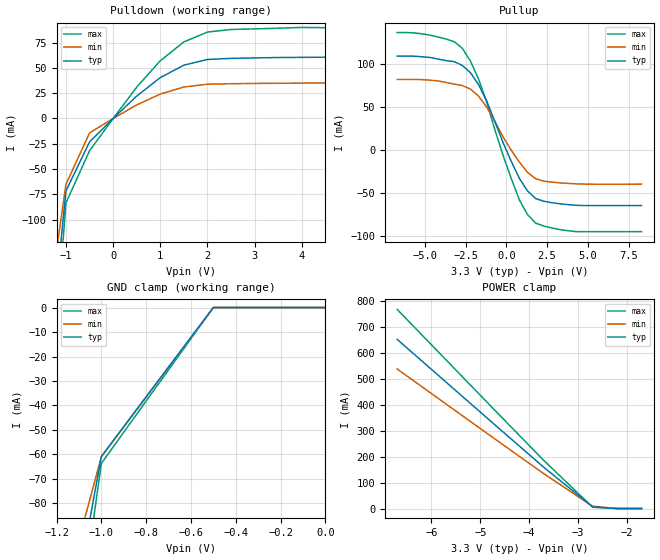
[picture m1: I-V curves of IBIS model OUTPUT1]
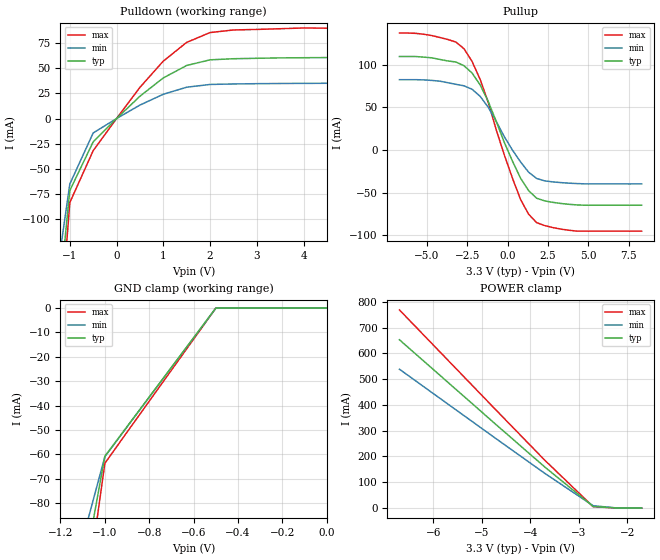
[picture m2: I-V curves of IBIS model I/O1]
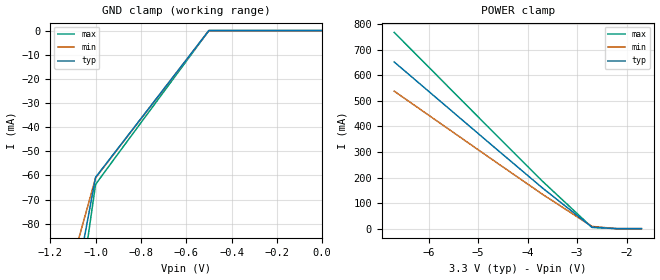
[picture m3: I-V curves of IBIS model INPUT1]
[IBIS Ver]   1.1
[File name]   960hxpq2.ibs
[File rev]   1.0
[Date]   5/10/96
[Source]   The file was oringinated at Intel Corporation.
[Notes]   The following information corresponds to the 80960HA
   in the 168 lead PGA package. This information has
   not been correlated to actual silicon.
[Disclaimer]   This information is for modeling purposes only and is
   not guaranteed.
[Component]   80960HX
[Manufacturer]  Intel
[Package]PQ@
|	typ   min   max
R_pkg	130m	117m	145m
L_pkg	12.4nH	10.9nH	13.9nH
C_pkg	1.1pF	.9pF	1.3pF
[Pin]   signal_name   model_name
A1	VSS		GND
A2	FAIL#		OUTPUT1
A3	DP0		I/O1
A4	DP2		I/O1
A5	VOLDET		OUTPUT1
A6	TRST		INPUT1
A7	TDI		INPUT1
A8	TDO		OUTPUT1
A9	NC		NC
A10	NC		NC
A11	CT0		OUTPUT1
A12	CT1		OUTPUT1
A13	CT2		OUTPUT1
A14	CT3		OUTPUT1
A15	XINT1#		INPUT1
A16	RESET#		RSTBUF
A17	XINT2#		INPUT1
B1	BOFF#		INPUT1
B2	STEST		INPUT1
B3	DP1		I/O1
B4	DP3		I/O1
B5	TCK		INPUT1
B6	TMS		INPUT1
B7	VCC		POWER
B8	PCHK#		OUTPUT1
B9	VCC		POWER
B10	VCCPLL		INPUT1
B11	VCC		POWER
B12	VCC		POWER
B13	NC		NC
B14	NC		NC
B15	XINT0#		INPUT1
B16	XINT3#		INPUT1
B17	XINT5#		INPUT1
C1	D3		I/O1
C2	D1		I/O1
C3	ONCE#		INPUT1
C4	VSS		GND
C5	VCC5		INPUT1
C6	VCC		POWER
C7	VSS		GND
C8	VSS		GND
C9	VSS		GND
C10	VSS		GND
C11	VSS		GND
C12	VSS		GND
C13	CLKIN		CLKBUF
C14	VSS		GND
C15	XINT4#		INPUT1
C16	XINT6#		INPUT1
C17	XINT7#		INPUT1
D1	D5		I/O1
D2	D2		I/O1
D3	NC		NC
D15	NMI#		INPUT1
D16	A2		OUTPUT1
D17	A3		OUTPUT1
E1	D7		I/O1
E2	D4		I/O1
E3	D0		I/O1
E15	VCC		POWER
E16	A4		OUTPUT1
E17	A5		OUTPUT1
F1	D8		I/O1
F2	D6		I/O1
F3	VCC		POWER
F15	VSS		GND
F16	VCC		POWER
F17	A6		OUTPUT1
G1	D9		I/O1
G2	VCC		POWER
G3	VSS		GND
G15	VSS		GND
G16	A7		OUTPUT1
G17	A8		OUTPUT1
H1	D11		I/O1
H2	D10		I/O1
H3	VSS		GND
H15	VSS		GND
H16	VCC		POWER
H17	A9		OUTPUT1
J1	D12		I/O1
J2	VCC		POWER
J3	VSS		GND
J15	VSS		GND
J16	VCC		POWER
J17	A10		OUTPUT1
K1	D13		I/O1
K2	VCC		POWER
K3	VSS		GND
K15	VSS		GND
K16	VCC		POWER
K17	A11		OUTPUT1
L1	D15		I/O1
L2	D14		I/O1
L3	VSS		GND
L15	VSS		GND
L16	A13		OUTPUT1
L17	A12		OUTPUT1
M1	D16		I/O1
M2	VCC		POWER
M3	VSS		GND
M15	VSS		GND
M16	VCC		POWER
M17	A14		OUTPUT1
N1	D17		I/O1
N2	D18		I/O1
N3	VCC		POWER
N15	VCC		POWER
N16	A16		OUTPUT1
N17	A15		OUTPUT1
P1	A19		OUTPUT1
P2	D20		I/O1
P3	D22		I/O1
P15	A20		OUTPUT1
P16	A19		OUTPUT1
P17	A17		OUTPUT1
Q1	D21		I/O1
Q2	D23		I/O1
Q3	D26		I/O1
Q4	D28		I/O1
Q5	D30		I/O1
Q6	VCC		POWER
Q7	VSS		GND
Q8	VSS		GND
Q9	VSS		GND
Q10	VSS		GND
Q11	VSS		GND
Q12	SUP#		OUTPUT1
Q13	A30		OUTPUT1
Q14	A28		OUTPUT1
Q15	A24		OUTPUT1
Q16	A21		OUTPUT1
Q17	A18		OUTPUT1
R1	D24		I/O1
R2	D27		I/O1
R3	D31		I/O1
R4	BTERM#		INPUT1
R5	HOLD		INPUT1
R6	ADS#		OUTPUT1
R7	VCC		POWER
R8	VCC		POWER
R9	BE0#		OUTPUT1
R10	VCC		POWER
R11	VCC		POWER
R12	BSTALL		OUTPUT1
R13	BREQ		OUTPUT1
R14	A29		OUTPUT1
R15	A26		OUTPUT1
R16	A23		OUTPUT1
R17	A22		OUTPUT1
S1	D25		I/O1
S2	D29		I/O1
S3	READY#		INPUT1
S4	HOLDA		OUTPUT1
S5	BE3#		OUTPUT1
S6	BE2#		OUTPUT1
S7	BE1#		OUTPUT1
S8	BLAST#		OUTPUT1
S9	DEN#		OUTPUT1
S10	W/R#		OUTPUT1
S11	DT#/R#		OUTPUT1
S12	WAIT#		OUTPUT1
S13	D#/C#		OUTPUT1
S14	LOCK#		OUTPUT1
S15	A31		OUTPUT1
S16	A27		OUTPUT1
S17	A25		OUTPUT1
| Models and submodels in the file (5): OUTPUT1 (Output), I/O1 (I/O), INPUT1 (Input), CLKBUF (Input), RSTBUF (Input)
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|This following model descriptions describe each of the
|different type of buffers.
|This is the model for buffer OUTPUT1.
[Model] OUTPUT1
Model_type Output
Polarity Non-Inverting
Enable Active-High
|signals  FAIL#,VOLDET,CT(3:0),PCHK#,A(31:2),SUP#,ADS#,BE(3:0)#,BSTALL,
|   BREQ,HOLDA,BLAST#,DEN#,W/R#,DT#/R#,WAIT#,D#/C#,LOCK#,TDO
|variable   typ   min   max
C_comp   3.2pf	2.9pf	3.5pf
|variable   typ   min   max
[Voltage range]   3.3V   3.0V   3.6V
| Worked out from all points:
|   slope of the pulldown table from 0 to 0.495 V, typ, clamps not added: 22.6 ohm
|   slope of the pullup table from 0 to 0.495 V, typ, clamps not added: 23.8 ohm
|   GND clamp passes 1 mA (typ) near -0.51 V on its own axis
|   POWER clamp passes 1 mA (typ) near -2.28 V on its own axis
[Pulldown]
|Voltage   I(typ)   I(min)   I(max)
-5V       -2.148A    -1.467A    -2.772A
-1.5V     -307.3mA   -227.6mA   -382.9mA
-1V       -71.49mA   -65.01mA   -83.39mA
-500mV    -23.17mA   -14.29mA   -31.92mA
500mV     22.15mA    13.38mA    30.94mA
1V        40.34mA    24.11mA    57.02mA
1.5V      52.68mA    31.12mA    75.61mA
2V        58.31mA    33.86mA    85.36mA
2.5V      59.38mA    34.34mA    87.93mA
4V        60.39mA    34.93mA    89.94mA
10V       60.77mA    35.16mA    90.06mA
|Note that the pullup voltage in the data table is derived from the
|equation:
|Vtable = Vcc - Voutput
|For the 8.3V in the table it is actually 8.3 volts below Vcc and
|-3.3V with respect to ground.
[Pullup]
|Voltage   I(typ)   I(min)   I(max)
-6.7V     109.6mA    82.49mA    137.1mA
-4.2V     106.2mA    80.75mA    131.9mA
-3.2V     103.2mA    77.06mA    126.5mA
-2.7V     98.79mA    75.33mA    118.7mA
-1.7V     76.29mA    62.98mA    82.73mA
-1.2V     57mA       50.13mA    55.93mA
-200mV    8.81mA     15.56mA    -5.959mA
800mV     -32.82mA   -13.78mA   -57.82mA
1.3V      -47.47mA   -25.86mA   -75.07mA
1.8V      -56.38mA   -33.22mA   -84.96mA
4.3V      -64.2mA    -39.19mA   -94.9mA
8.3V      -64.54mA   -39.59mA   -94.91mA
[GND_Clamp]
|Voltage   I(typ)   I(min)   I(max)
-5V       -2.148A    -1.466A    -2.772A
-2V       -564.4mA   -400.4mA   -716.6mA
-1V       -60.81mA   -61.01mA   -63.72mA
-900mV    -48.65mA   -48.79mA   -50.93mA
-800mV    -36.49mA   -36.6mA    -38.2mA
-700mV    -24.32mA   -24.4mA    -25.46mA
-600mV    -12.16mA   -12.2mA    -12.73mA
-500mV    0A         0A         0A
-400mV    0A         0A         0A
0V        0A         0A         0A
|Note that the voltages in the Power_clamp data table are Vcc relative
|which means they are referenced to Vcc.  The voltages in the table are
|derived from the following equation:
|Vtable = Vcc - Voutput
|0V in the table is actually 3.3V with respect to ground and 0V above Vcc.
[POWER_Clamp]
|Voltage   I(typ)   I(min)   I(max)
-6.7V     652.6mA    538.3mA    768.3mA
-4.7V     322.7mA    268.2mA    378.8mA
-3.7V     159.1mA    134.5mA    185.5mA
-2.7V     6mA        8.856mA    4.991mA
-2.6V     4.8mA      7.109mA    3.988mA
-2.5V     3.6mA      5.338mA    2.997mA
-2.4V     2.4mA      3.559mA    1.994mA
-2.3V     1.2mA      1.779mA    1.003mA
-2.2V     0A         0A         0A
-1.7V     0A         0A         0A
[Ramp]
|   typ   min   max
dV/dt_r   1.3/0.3n	1.1/0.5n	1.5/0.3n
dV/dt_f		1.3/0.3n	1.0/0.5n	1.5/0.3n
|end of OUTPUT1 model
|This is the model for the buffer I/O1.
[Model] I/O1
Model_type I/O
Polarity Non-Inverting
Enable Active-High
|Signals  D(31:0),DP(3:0)
Vinl = 0.8V
Vinh = 2.0V
|variable   typ   min   max
C_comp   3.2pf	2.9pf	3.5pf
|variable   typ   min   max
[Voltage range]   3.3V   3.0V   3.6V
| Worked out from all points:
|   slope of the pulldown table from 0 to 0.495 V, typ, clamps not added: 22.6 ohm
|   slope of the pullup table from 0 to 0.495 V, typ, clamps not added: 23.8 ohm
|   GND clamp passes 1 mA (typ) near -0.51 V on its own axis
|   POWER clamp passes 1 mA (typ) near -2.28 V on its own axis
[Pulldown]
|Voltage   I(typ)   I(min)   I(max)
-5V       -2.148A    -1.467A    -2.772A
-1.5V     -307.3mA   -227.6mA   -382.9mA
-1V       -71.49mA   -65.01mA   -83.39mA
-500mV    -23.17mA   -14.29mA   -31.92mA
500mV     22.15mA    13.38mA    30.94mA
1V        40.34mA    24.11mA    57.02mA
1.5V      52.68mA    31.12mA    75.61mA
2V        58.31mA    33.86mA    85.36mA
2.5V      59.38mA    34.34mA    87.93mA
4V        60.39mA    34.93mA    89.94mA
10V       60.77mA    35.16mA    90.06mA
|Note that the pullup voltage in the data table is derived from the
|equation:
|Vtable = Vcc - Voutput
|For the 8.3V in the table it is actually 8.3 volts below Vcc and
|-3.3V with respect to ground.
[Pullup]
|Voltage   I(typ)   I(min)   I(max)
-6.7V     109.6mA    82.49mA    137.1mA
-4.2V     106.2mA    80.75mA    131.9mA
-3.2V     103.2mA    77.06mA    126.5mA
-2.7V     98.79mA    75.33mA    118.7mA
-1.7V     76.29mA    62.98mA    82.73mA
-1.2V     57mA       50.13mA    55.93mA
-200mV    8.81mA     15.56mA    -5.959mA
800mV     -32.82mA   -13.78mA   -57.82mA
1.3V      -47.47mA   -25.86mA   -75.07mA
1.8V      -56.38mA   -33.22mA   -84.96mA
4.3V      -64.2mA    -39.19mA   -94.9mA
8.3V      -64.54mA   -39.59mA   -94.91mA
[GND_Clamp]
|Voltage   I(typ)   I(min)   I(max)
-5V       -2.148A    -1.466A    -2.772A
-2V       -564.4mA   -400.4mA   -716.6mA
-1V       -60.81mA   -61.01mA   -63.72mA
-900mV    -48.65mA   -48.79mA   -50.93mA
-800mV    -36.49mA   -36.6mA    -38.2mA
-700mV    -24.32mA   -24.4mA    -25.46mA
-600mV    -12.16mA   -12.2mA    -12.73mA
-500mV    0A         0A         0A
-400mV    0A         0A         0A
0V        0A         0A         0A
|Note that the voltages in the Power_clamp data table are Vcc relative
|which means they are referenced to Vcc.  The voltages in the table are
|derived from the following equation:
|Vtable = Vcc - Voutput
|0V in the table is actually 3.3V with respect to ground and 0V above Vcc.
[POWER_Clamp]
|Voltage   I(typ)   I(min)   I(max)
-6.7V     652.6mA    538.3mA    768.3mA
-4.7V     322.7mA    268.2mA    378.8mA
-3.7V     159.1mA    134.5mA    185.5mA
-2.7V     6mA        8.856mA    4.991mA
-2.6V     4.8mA      7.109mA    3.988mA
-2.5V     3.6mA      5.338mA    2.997mA
-2.4V     2.4mA      3.559mA    1.994mA
-2.3V     1.2mA      1.779mA    1.003mA
-2.2V     0A         0A         0A
-1.7V     0A         0A         0A
[Ramp]
|   typ   min   max
dV/dt_r   1.3/0.3n	1.1/0.5n	1.5/0.3n
dV/dt_f		1.3/0.3n	1.0/0.5n	1.5/0.3n
|end of I/O1 model
|This is the model for the buffer INPUT1.
[Model] INPUT1
Model_type Input
Polarity Non-Inverting
Enable Active-High
|Signals  TRST,TDI,XINT(7:0)#,BOFF#,STEST,TCK,TMS,VCCPLL,ONCE#,
|	  VCC5,NMI#,BTERM#,HOLD,READY#
Vinl = 0.8V
Vinh = 2.0V
|variable   typ   min   max
C_comp   3.2pf	2.9pf	3.5pf
|variable   typ   min   max
[Voltage range]   3.3V   3.0V   3.6V
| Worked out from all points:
|   GND clamp passes 1 mA (typ) near -0.51 V on its own axis
|   POWER clamp passes 1 mA (typ) near -2.28 V on its own axis
[GND_Clamp]
|Voltage   I(typ)   I(min)   I(max)
-5V       -2.148A    -1.466A    -2.772A
-2V       -564.4mA   -400.4mA   -716.6mA
-1V       -60.81mA   -61.01mA   -63.72mA
-900mV    -48.65mA   -48.79mA   -50.93mA
-800mV    -36.49mA   -36.6mA    -38.2mA
-700mV    -24.32mA   -24.4mA    -25.46mA
-600mV    -12.16mA   -12.2mA    -12.73mA
-500mV    0A         0A         0A
-400mV    0A         0A         0A
0V        0A         0A         0A
|Note that the voltages in the Power_clamp data table are Vcc relative
|which means they are referenced to Vcc.  The voltages in the table are
|derived from the following equation:
|Vtable = Vcc - Voutput
|0V in the table is actually 3.3V with respect to ground and 0V above Vcc.
[POWER_Clamp]
|Voltage   I(typ)   I(min)   I(max)
-6.7V     652.6mA    538.3mA    768.3mA
-4.7V     322.7mA    268.2mA    378.8mA
-3.7V     159.1mA    134.5mA    185.5mA
-2.7V     6mA        8.856mA    4.991mA
-2.6V     4.8mA      7.109mA    3.988mA
-2.5V     3.6mA      5.338mA    2.997mA
-2.4V     2.4mA      3.559mA    1.994mA
-2.3V     1.2mA      1.779mA    1.003mA
-2.2V     0A         0A         0A
-1.7V     0A         0A         0A
